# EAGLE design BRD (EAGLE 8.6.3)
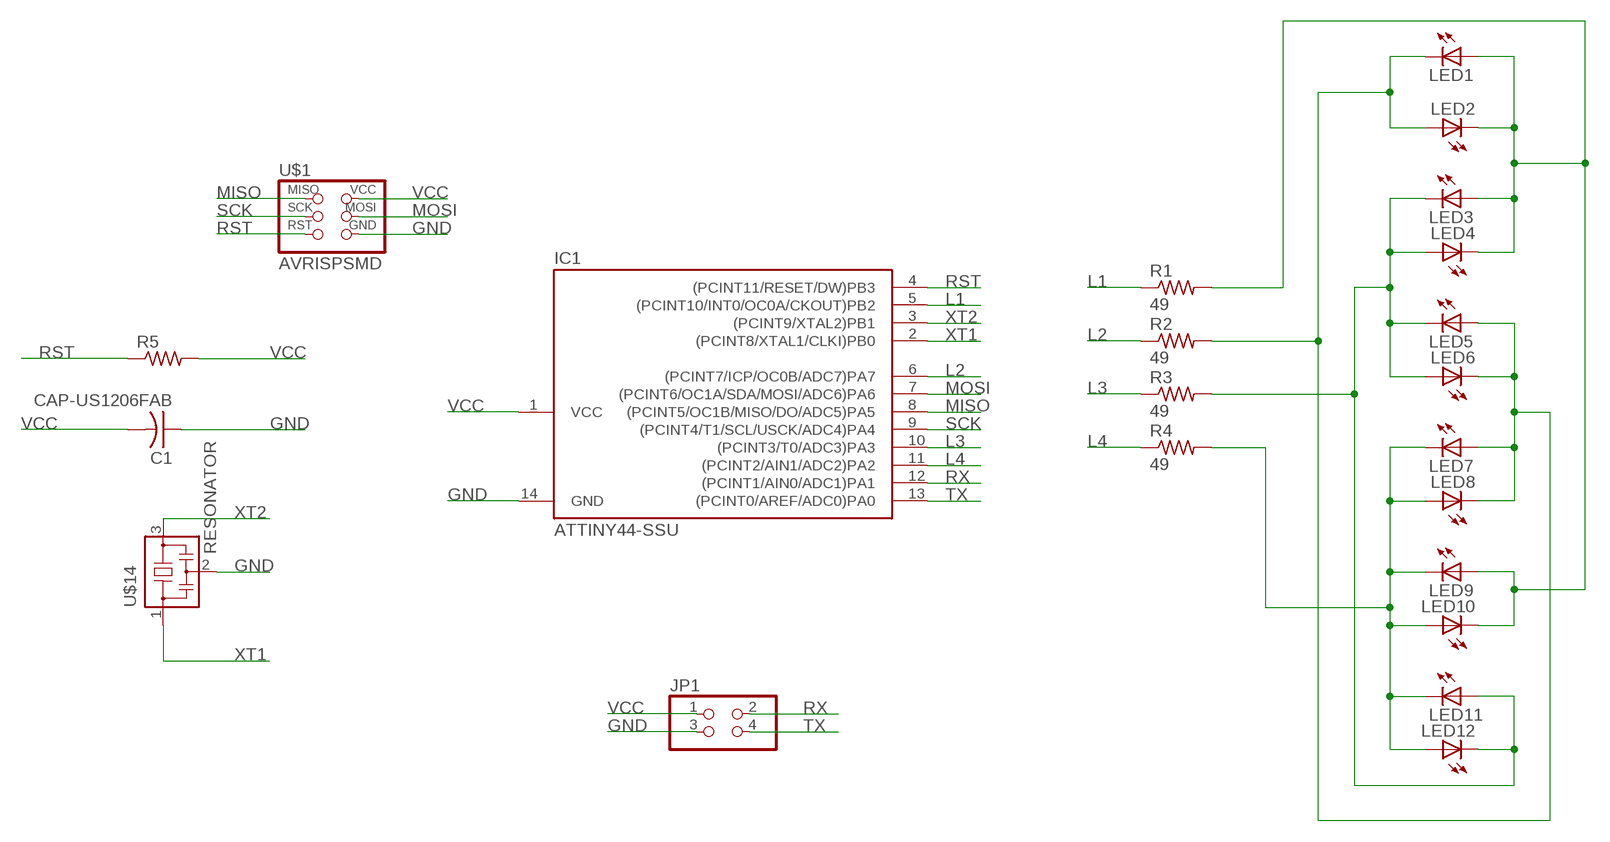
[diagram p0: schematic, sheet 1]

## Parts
C1  CAP-US1206FAB  [C1206FAB]
IC1  ATTINY44-SSU  [SOIC14]
JP1  PINHD-2X2  [2X02]
LED1  LEDFAB1206  [LED1206FAB]
LED2  LEDFAB1206  [LED1206FAB]
LED3  LEDFAB1206  [LED1206FAB]
LED4  LEDFAB1206  [LED1206FAB]
LED5  LEDFAB1206  [LED1206FAB]
LED6  LEDFAB1206  [LED1206FAB]
LED7  LEDFAB1206  [LED1206FAB]
LED8  LEDFAB1206  [LED1206FAB]
LED9  LEDFAB1206  [LED1206FAB]
LED10  LEDFAB1206  [LED1206FAB]
LED11  LEDFAB1206  [LED1206FAB]
LED12  LEDFAB1206  [LED1206FAB]
R1  49  RES-US1206FAB  [R1206FAB]
R2  49  RES-US1206FAB  [R1206FAB]
R3  49  RES-US1206FAB  [R1206FAB]
R4  49  RES-US1206FAB  [R1206FAB]
R5  RES-US1206FAB  [R1206FAB]
U$1  AVRISPSMD  [2X03SMD]
U$14  RESONATOR  [EFOBM]

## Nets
GND: C1.1 IC1.14(GND) JP1.3 U$1.6(GND) U$14.2
L1: IC1.5((PCINT10/INT0/OC0A/CKOUT)PB2) R1.1
L2: IC1.6((PCINT7/ICP/OC0B/ADC7)PA7) R2.1
L3: IC1.10((PCINT3/T0/ADC3)PA3) R3.1
L4: IC1.11((PCINT2/AIN1/ADC2)PA2) R4.1
MISO: IC1.8((PCINT5/OC1B/MISO/DO/ADC5)PA5) U$1.1(MISO)
MOSI: IC1.7((PCINT6/OC1A/SDA/MOSI/ADC6)PA6) U$1.4(MOSI)
N$1: LED1.1(A) LED2.2(C) LED3.1(A) LED4.2(C) LED9.1(A) LED10.2(C) R1.2
N$2: LED1.2(C) LED2.1(A) LED5.1(A) LED6.2(C) LED7.1(A) LED8.2(C) R2.2
N$5: LED3.2(C) LED4.1(A) LED5.2(C) LED6.1(A) LED11.1(A) LED12.2(C) R3.2
N$7: LED7.2(C) LED8.1(A) LED9.2(C) LED10.1(A) LED11.2(C) LED12.1(A) R4.2
RST: IC1.4((PCINT11/RESET/DW)PB3) R5.1 U$1.5(RST)
RX: IC1.12((PCINT1/AIN0/ADC1)PA1) JP1.2
SCK: IC1.9((PCINT4/T1/SCL/USCK/ADC4)PA4) U$1.3(SCK)
TX: IC1.13((PCINT0/AREF/ADC0)PA0) JP1.4
VCC: C1.2 IC1.1(VCC) JP1.1 R5.2 U$1.2(VCC)
XT1: IC1.2((PCINT8/XTAL1/CLKI)PB0) U$14.1
XT2: IC1.3((PCINT9/XTAL2)PB1) U$14.3

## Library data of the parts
C1 = fab:CAP-US
IC1 = fab:ATTINY44
JP1 = pinhead:PINHD-2X2: PIN HEADER
LED1-LED12 = fab:LED: LED
R1-R5 = fab:RES-US: Resistor (US Symbol)
U$1 = fab:AVRISP
U$14 = fab:RESONATOR

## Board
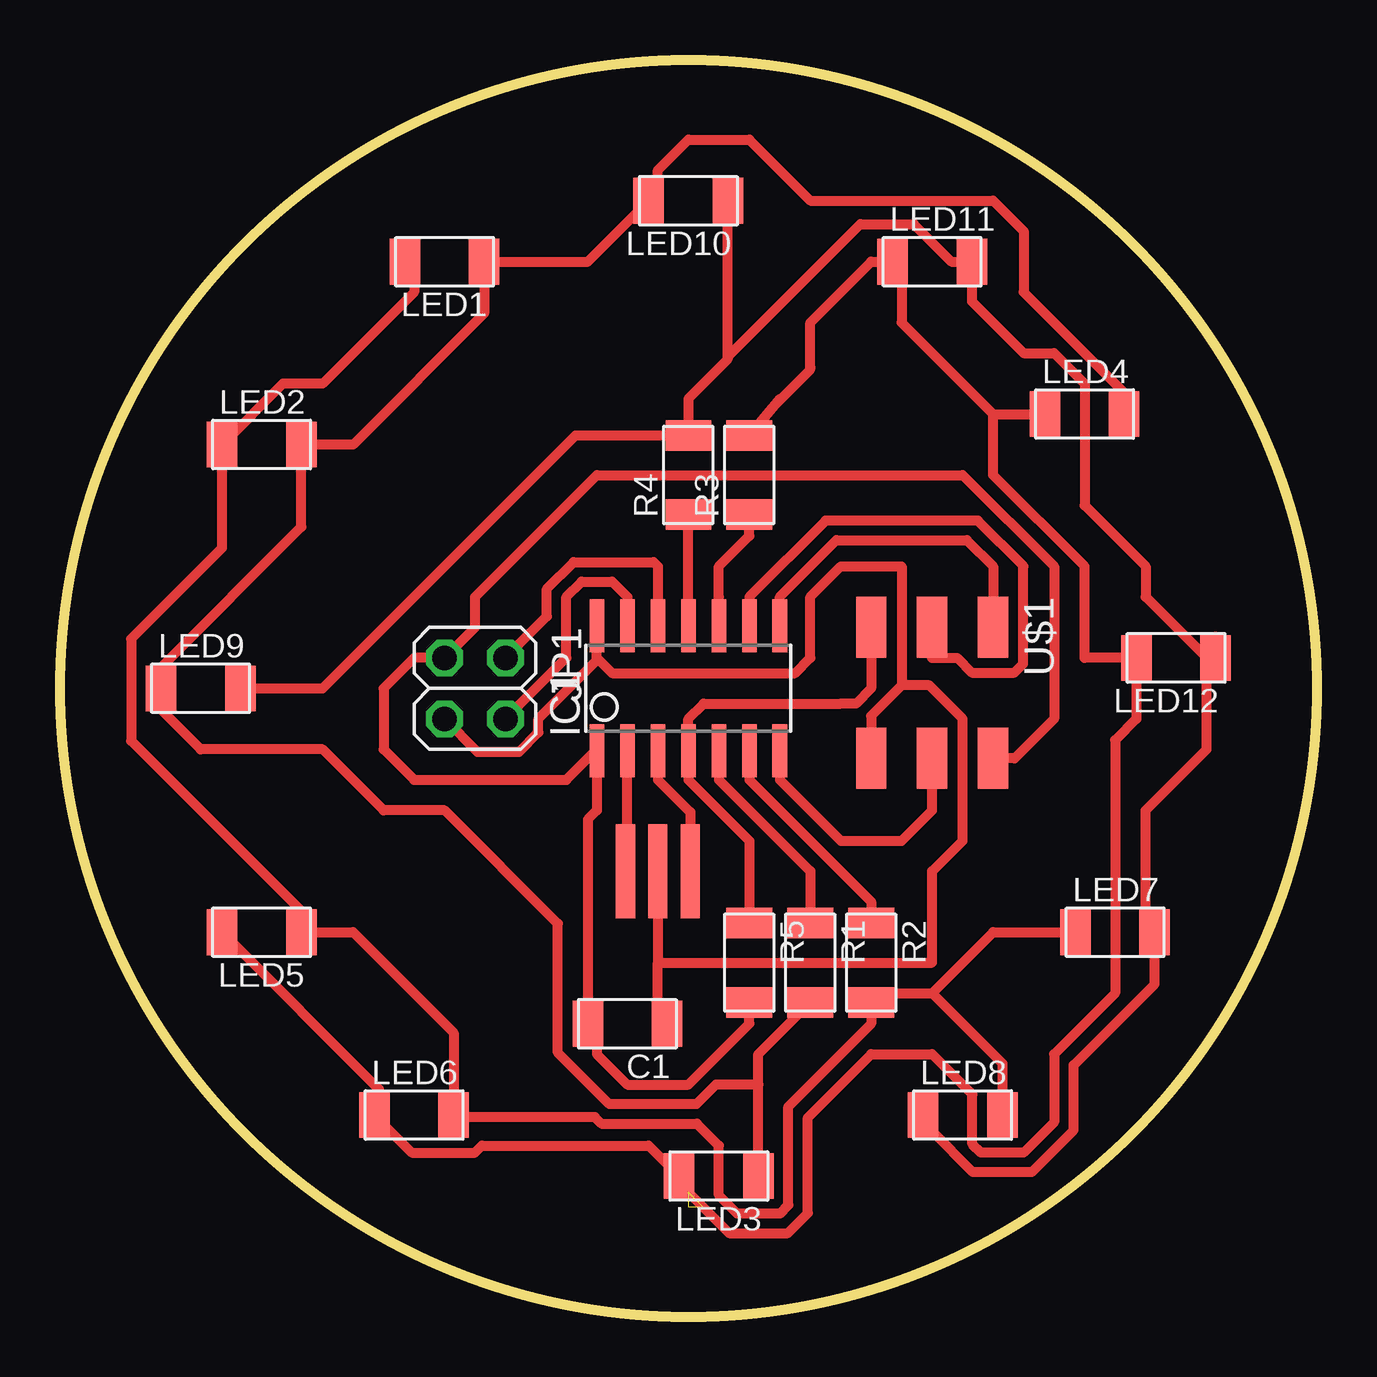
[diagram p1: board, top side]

Size 52.36 x 52.36 mm. Coordinates in mm from the lower left corner, seen from the top.
Outline: circle at 26.18,26.18 radius 26.18
Copper layers (1*16): Top 0.035mm / dielectric 1.5mm / Bottom 0.035mm
Design rules "default *": minimum track width 16mil, minimum drill 0.35mm, track to track 16mil, track to pad 16mil, pad to pad 16mil, via to via 16mil, smd to smd 16mil, copper to edge 16mil, drill to drill 16mil, minimum pad ring 10mil, minimum via ring 8mil, stop-mask expansion 4mil, vias tented up to drill 0mil, thermal gap 10mil

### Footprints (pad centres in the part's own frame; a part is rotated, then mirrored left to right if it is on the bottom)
C1206FAB = smd 1.27 x 1.905: 1 -1.651,0; 2 1.651,0
SOIC14 = smd 0.61 x 2.21: 1 -3.81,-2.603; 2 -2.54,-2.603; 3 -1.27,-2.603; 4 0,-2.603; 5 1.27,-2.603; 6 2.54,-2.603; 7 3.81,-2.603; 8 3.81,2.603; 9 2.54,2.603; 10 1.27,2.603; 11 0,2.603; 12 -1.27,2.603; 13 -2.54,2.603; 14 -3.81,2.603
2X02 = drill 1.016 octagon: 1 -1.27,-1.27; 2 -1.27,1.27; 3 1.27,-1.27; 4 1.27,1.27
LED1206FAB = smd 1.27 x 1.905: 1 -1.651,0; 2 1.651,0
R1206FAB = smd 1.27 x 1.905: 1 -1.651,0; 2 1.651,0
2X03SMD = smd 2.54 x 1.27: 1 -2.54,2.54; 2 2.92,2.54; 3 -2.54,0; 4 2.92,0; 5 -2.54,-2.54; 6 2.92,-2.54
EFOBM = smd 0.8 x 3.9: 1 -1.35,0; 2 0,0; 3 1.35,0

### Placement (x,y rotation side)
C1  23.64,12.21 180 top
IC1  26.18,26.18 0 top
JP1  17.29,26.18 270 top
LED1  16.02,43.96 180 top
LED2  8.4,36.34 0 top
LED3  27.45,5.86 180 top
LED4  42.69,37.61 0 top
LED5  8.4,16.02 180 top
LED6  14.75,8.4 0 top
LED7  43.96,16.02 0 top
LED8  37.61,8.4 0 top
LED9  5.86,26.18 0 top
LED10  26.18,46.5 180 top
LED11  36.34,43.96 0 top
LED12  46.5,27.45 180 top
R1  31.26,14.75 270 top
R2  33.8,14.75 270 top
R3  28.72,35.07 90 top
R4  26.18,35.07 90 top
R5  28.72,14.75 270 top
U$1  36.34,26.18 270 top
U$14  24.91,18.56 0 top

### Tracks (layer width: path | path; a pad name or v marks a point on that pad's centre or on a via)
GND
  Top 0.406: 22.37,28.72 IC1.14 22.37,27.45 | U$14.2 24.91,14.75 | 22.37,27.45 23.01,26.82 30.63,26.82 31.26,27.45 31.26,29.99 32.53,31.26 35.07,31.26 35.07,26.3 | JP1.3 17.39,23.54 19.13,23.54 19.93,24.34 19.93,24.91 22.37,27.35 22.37,27.45 | 24.91,14.75 36.34,14.75 36.34,18.56 37.61,19.83 37.61,24.91 36.22,26.3 35.07,26.3 | C1.1 24.91,12.59 24.91,14.75 | 35.07,26.3 33.8,25.03 U$1.6
L1
  Top 0.406: IC1.5 27.45,22.37 31.26,18.56 R1.1
L2
  Top 0.406: IC1.6 28.72,22.37 33.8,17.29 R2.1
L3
  Top 0.406: 27.45,29.99 IC1.10 27.45,31.26 28.72,32.53 R3.1
L4
  Top 0.406: IC1.11 R4.1
MISO
  Top 0.406: 29.99,29.36 IC1.8 29.99,29.99 32.35,32.35 37.79,32.35 38.88,31.26 U$1.1
MOSI
  Top 0.406: 29.99,23.01 IC1.7 29.99,22.37 32.53,19.83 35.07,19.83 36.34,21.1 U$1.4
N$1
  Top 0.406: LED4.2 44.34,38.5 40.15,42.69 40.15,45.23 38.88,46.5 31.26,46.5 28.72,49.04 26.18,49.04 24.91,47.77 24.91,46.88 LED10.2 21.99,43.96 LED1.1 17.67,41.8 12.21,36.34 LED2.2 10.05,32.91 4.21,27.07 LED9.1 | R1.2 29.1,10.94 29.1,9.67 | LED3.1 29.1,9.67 | 29.1,9.67 27.33,9.67 26.52,8.86 22.89,8.86 20.75,11.01 20.75,16.38 16.02,21.1 13.48,21.1 10.94,23.64 5.86,23.64 4.21,25.29 LED9.1 | LED9.1 4.59,26.56
N$2
  Top 0.406: 36.34,13.48 34.18,13.48 R2.2 33.8,12.21 30.35,8.76 30.35,4.66 29.99,4.3 28.21,4.3 27.45,5.06 27.45,7.13 26.54,8.05 22.56,8.05 22.29,8.32 16.49,8.32 LED6.2 16.4,11.83 12.21,16.02 LED5.1 10.05,16.91 2.97,24 2.97,28.25 6.75,32.03 LED2.1 9.29,38.88 10.94,38.88 14.75,42.69 14.75,43.58 LED1.2 | LED7.1 38.88,16.02 36.34,13.48 | LED8.2 39.26,10.56 36.34,13.48
N$5  (3 unrouted)
  Top 0.406: 29.99,38.25 29.68,37.87 | 29.68,37.87 R3.2 | 29.68,37.87 31.19,39.38 arc45 31.26,39.56 31.26,41.42 33.8,43.96 LED11.1 35.07,43.58 35.07,41.42 38.88,37.61 | 38.88,37.61 LED4.1 | 38.88,37.61 38.88,35.07 42.69,31.26 42.69,27.45 LED12.2 44.85,24.91 43.96,24.02 43.96,13.48 41.42,10.94 41.42,8.11 40.15,6.84 38.37,6.84 38.02,7.2 38.02,9.27 36.34,10.94 33.8,10.94 31.16,8.3 31.16,4.32 30.33,3.49 27.88,3.49 26.18,5.18 26.18,5.48 LED3.2 24.53,7.13 17.58,7.13 17.29,6.84 14.66,6.84 13.29,8.21 | LED6.1 13.29,8.21 | LED5.2 13.29,9.48 13.29,8.21
N$7
  Top 0.406: 27.83,40 arc-45 27.76,39.82 26.18,38.25 R4.2 21.48,36.72 10.94,26.18 LED9.2 | 27.83,40 LED10.1 | 48.15,28.34 LED12.1 47.77,27.45 | 47.77,27.45 45.23,29.99 45.23,31.26 42.69,33.8 42.69,38.88 41.42,40.15 40.15,40.15 37.99,42.31 LED11.2 37.14,43.96 35.58,45.52 33.35,45.52 27.83,40 | 47.77,27.45 47.77,23.64 45.23,21.1 45.23,16.4 LED7.2 45.61,13.86 42.23,10.48 42.23,7.77 40.49,6.03 38.04,6.03 36.34,7.72 36.34,8.02 LED8.1
RST
  Top 0.406: R5.1 28.72,19.83 26.18,22.37 IC1.4 26.18,24.91 26.82,25.55 32.53,25.55 33.17,25.55 33.8,26.18 U$1.5
RX
  Top 0.406: JP1.2 20.29,29.18 20.29,30.33 21.4,31.44 24.73,31.44 24.91,31.26 IC1.12
SCK
  Top 0.406: IC1.9 28.72,29.99 31.9,33.17 38.25,33.17 40.15,31.26 40.13,31.24 40.13,27.2 39.77,26.84 37.99,26.84 37.38,27.45 36.34,27.45 U$1.3
TX
  Top 0.406: IC1.13 23.64,29.99 23.01,30.63 21.74,30.63 21.1,29.99 21.1,27.45 JP1.4
VCC
  Top 0.406: R5.2 28.72,12.21 26.18,9.67 23.64,9.67 22.37,10.94 22.37,11.83 C1.2 21.99,20.72 22.37,21.1 IC1.1 22.31,23.58 21.1,22.37 14.75,22.37 13.48,23.64 13.48,26.18 14.75,27.45 JP1.1 17.29,28.72 17.29,29.99 22.37,35.07 37.61,35.07 41.42,31.26 41.42,24.91 39.77,23.26 U$1.2
XT1
  Top 0.406: U$14.1 23.64,18.64 IC1.2
XT2
  Top 0.406: 26.18,17.29 U$14.3 26.26,21.02 24.91,22.37 IC1.3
